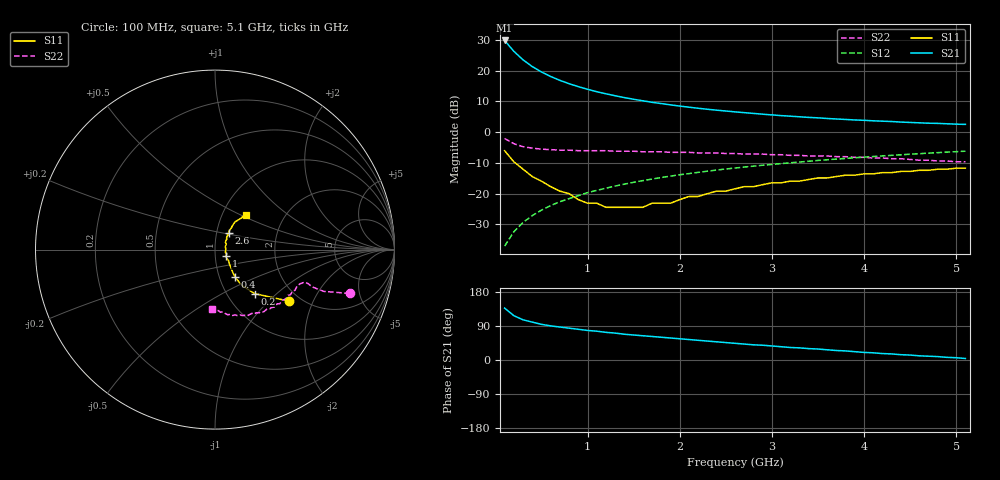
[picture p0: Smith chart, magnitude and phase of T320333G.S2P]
!AT-32033
!S and NOISE PARAMETERS at Vce=2.7V  Ic=20mA.  LAST UPDATED 01-05-95
# ghz s ma r 50
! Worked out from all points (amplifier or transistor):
!   51 points, 100 MHz to 5.1 GHz, reference 50 ohm
!   highest |S21| = 29.8 dB at 100 MHz (marker M1)
!   |S21| within 3 dB of that: start of sweep to 185.1 MHz
!   unconditionally stable (mu >= 1): 665.4 MHz to 2.273 GHz
!   at 900 MHz: K = 1.02, MAG = 16.9 dB, |S12| = -20.6 dB
!   at 2.6 GHz: K = 0.99, MSG = 9.1 dB, |S12| = -11.7 dB
!   at 5.1 GHz: K = 0.94, MSG = 4.4 dB, |S12| = -6.2 dB
!   S11 on the Smith chart (normalised r, x): 100 MHz: 1.74, -1.33; 200 MHz: 1.34, -0.74; 400 MHz: 1.19, -0.38; 1 GHz: 1.12, -0.08; 2.6 GHz: 1.14, +0.22; 5.1 GHz: 1.30, +0.54
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0.1  0.5 -35.0  31.03 137.0  0.014 77.0  0.79 -18.0
0.2  0.33 -48.0  20.68 117.0  0.024 76.0  0.65 -21.0
0.3  0.25 -53.0  15 106.0  0.034 76.0  0.58 -21.0
0.4  0.19 -54.0  11.67 100.0  0.044 77.0  0.55 -20.0
0.5  0.16 -52.0  9.53 94.0  0.054 77.0  0.53 -20.0
0.6  0.13 -48.0  8.05 90.0  0.064 76.0  0.52 -21.0
0.7  0.11 -44.0  6.96 87.0  0.074 76.0  0.51 -22.0
0.8  0.1 -40.0  6.15 84.0  0.083 75.0  0.51 -22.0
0.9  0.08 -36.0  5.5 81.0  0.093 75.0  0.5 -24.0
1  0.07 -31.0  4.99 78.0  0.104 74.0  0.5 -25.0
1.1  0.07 -20.0  4.55 76.0  0.113 73.0  0.5 -26.0
1.2  0.06 -16.0  4.21 73.0  0.123 72.0  0.5 -27.0
1.4  0.06 3.0  3.65 68.0  0.143 70.0  0.49 -30.0
1.6  0.06 17.0  3.24 64.0  0.163 68.0  0.48 -32.0
1.8  0.07 31.0  2.92 60.0  0.183 66.0  0.48 -35.0
2.2  0.09 45.0  2.45 52.0  0.222 61.0  0.46 -41.0
2.6  0.12 51.0  2.14 44.0  0.261 57.0  0.45 -47.0
3.2  0.16 53.0  1.82 33.0  0.318 50.0  0.42 -57.0
3.5  0.18 54.0  1.71 29.0  0.347 46.0  0.41 -62.0
4  0.21 52.0  1.56 20.0  0.393 41.0  0.39 -71.0
4.3  0.22 51.0  1.49 16.0  0.42 37.0  0.37 -77.0
5.1  0.26 48.0  1.34 4.0  0.491 28.0  0.33 -93.0
